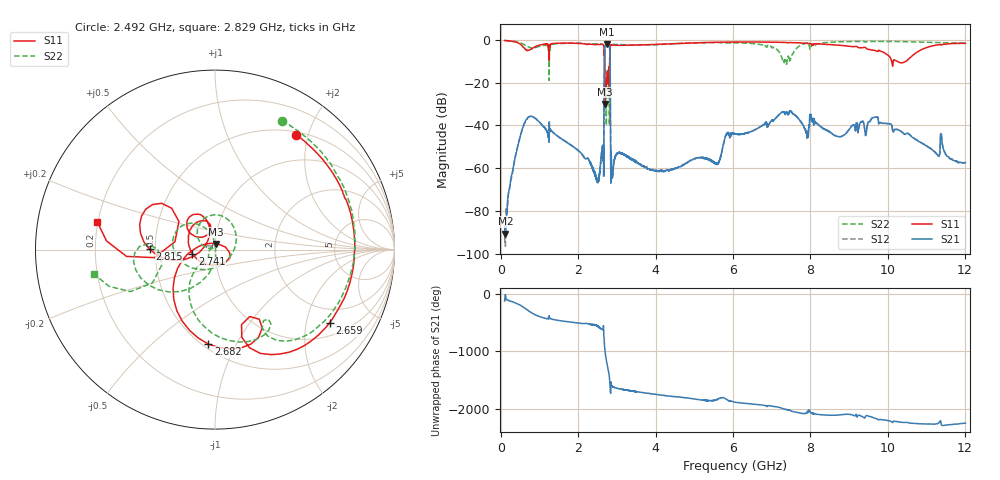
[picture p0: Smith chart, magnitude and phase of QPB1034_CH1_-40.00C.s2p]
! TDS: k:\Engsetup\Winsaw\QPB1034_ALL
! Channel 1
! Ports=1 2
! seg 1=100.000000 1100.000000 51
! seg 2=1101.000000 1301.000000 201
! seg 3=1302.000000 2302.000000 101
! seg 4=2303.000000 3503.000000 1201
! seg 5=3504.000000 5204.000000 171
! seg 6=5205.000000 6405.000000 1201
! seg 7=6406.000000 8506.000000 211
! seg 8=8507.000000 12007.000000 176
! Points=3313
! FailCode=0
! Topology=ALL_SE(12)
!VNA Cal loaded =QPB1034_ALL_-40C
!PS1(V)= 5.000
!PS(mA)= 0.192
!PS2(V)= 0.630
!PS(mA)= -0.001
!PS3(V)= 0.630
!PS(mA)= 0.000
!PS4(V)= 1.170
!PS(mA)= -0.001
!Temp (C)= -40.00
# MHz S DB R 50
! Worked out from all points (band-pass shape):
!   3313 points, 100 MHz to 12.01 GHz, reference 50 ohm
!   highest |S21| = -2.05 dB at 2.734 GHz (marker M1); lowest = -90.6 dB at 120 MHz (marker M2)
!   |S21| within 3 dB of the highest: 2.688 GHz to 2.818 GHz (130.5 MHz wide, 4.74 % of centre)
!   lowest |S11| = -30.0 dB at 2.697 GHz (marker M3), VSWR 1.07, Z = 50.2 + j3.16 ohm
!   |S11| at or under -10 dB: 2.688 GHz to 2.814 GHz (125.8 MHz wide, 4.57 % of centre); 10.10077 GHz to 10.14308 GHz (42.31 MHz wide, 0.418 % of centre); 10.24 GHz to 10.47 GHz (228.7 MHz wide, 2.21 % of centre)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
!   |S22| runs from -40.1 to -0.3 dB; largest |S21 - S12| = 0.0043
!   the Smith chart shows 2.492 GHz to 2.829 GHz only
!   S11 on the Smith chart (normalised r, x): 2.492 GHz: 0.54, +1.80; 2.659 GHz: 1.43, -2.75; 2.682 GHz: 0.53, -0.78; 2.741 GHz: 0.78, -0.04; 2.815 GHz: 0.47, +0.00; 2.829 GHz: 0.20, +0.11
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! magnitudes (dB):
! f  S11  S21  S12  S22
! 100 MHz  -0.3  -86.9  -92.3  -0.3
! 120 MHz  -0.3  -90.6  -96.5  -0.3
! 240 MHz  -0.5  -67.8  -68.4  -0.5
! 500 MHz  -1.9  -45.2  -45.2  -1.3
! 1.1 GHz  -2.0  -40.4  -40.4  -2.6
! 2.434 GHz  -2.2  -62.8  -63.2  -1.9
! 2.492 GHz  -2.1  -65.3  -65.0  -1.9
! 2.659 GHz  -2.4  -57.3  -57.3  -2.5
! 2.682 GHz  -5.6  -7.8  -7.8  -5.8
! 2.697 GHz  -30.0  -3.0  -3.0  -20.7
! 2.717 GHz  -20.7  -2.3  -2.3  -31.6
! 2.734 GHz  -20.1  -2.0  -2.0  -28.8
! 2.741 GHz  -17.9  -2.1  -2.1  -20.6
! 2.815 GHz  -8.8  -4.0  -4.0  -9.2
! 2.829 GHz  -3.4  -15.2  -15.3  -3.3
! 2.853 GHz  -2.4  -52.5  -52.4  -2.1
! 2.883 GHz  -2.4  -64.0  -64.7  -2.1
! 3.054 GHz  -2.5  -52.9  -52.8  -2.2
! 5.406 GHz  -1.2  -56.2  -56.3  -1.2
! 7.376 GHz  -1.2  -33.9  -33.8  -10.3
! 9.807 GHz  -5.2  -38.6  -38.6  -0.7
! 12.01 GHz  -1.6  -57.6  -57.3  -1.4
